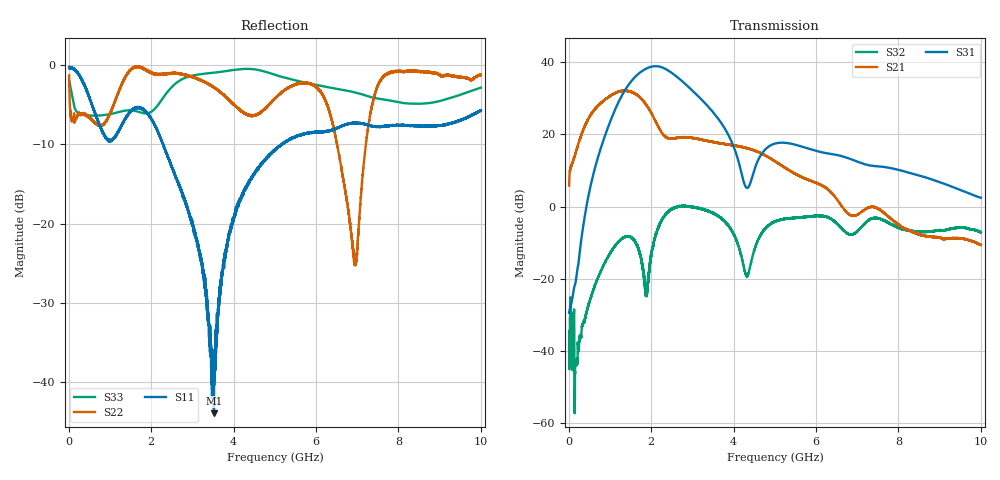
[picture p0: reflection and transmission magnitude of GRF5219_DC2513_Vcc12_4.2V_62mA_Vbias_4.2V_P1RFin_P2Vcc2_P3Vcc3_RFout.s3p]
!Keysight Technologies,N5245B,MY56052315,A.20.20.05
!Date: Friday, August 21, 2026 15:38:49
!Correction: S11(C  3-Port  )
!S12(C  3-Port  )
!S13(C  3-Port  )
!S21(C  3-Port  )
!S22(C  3-Port  )
!S23(C  3-Port  )
!S31(C  3-Port  )
!S32(C  3-Port  )
!S33(C  3-Port  )
!S3P File: Measurements: <S11,S12,S13>,
!<S21,S22,S23>,
!<S31,S32,S33>:
# Hz S  dB  R 50
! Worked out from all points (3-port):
!   9991 points, 10 MHz to 10 GHz, reference 50 ohm
!   strongest paths, dB at 10 MHz, 2.507 GHz, 5.005 GHz, 7.503 GHz, 10 GHz:
!     S31: -29.5, 37.0, 17.4, 11.1, 2.4
!     S21: 5.8, 18.8, 12.5, -0.6, -10.6
!     S32: -39.1, -0.7, -4.1, -3.2, -7.2
!   lowest |S11| = -43.9 dB at 3.524 GHz (marker M1), VSWR 1.01, Z = 49.9 - j0.623 ohm
!   |S11| at or under -10 dB: 2.290023 GHz to 2.292511 GHz (2.488 MHz wide, 0.109 % of centre); 2.293 GHz to 5.161 GHz (2.867 GHz wide, 76.9 % of centre); 5.161129 GHz to 5.16885 GHz (7.721 MHz wide, 0.149 % of centre)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
1e7  -0.37 -2.0  -54.46 -16.0  -63.07 72.6
     5.79 74.4  -1.31 -49.6  -58.02 113.3
     -29.47 -170.9  -39.08 7.9  -1.92 -57.0
6.06e8  -5.67 -92.1  -41.03 102.5  -66.14 110.3
        26.48 26.3  -7.09 169.1  -43.30 -64.5
        9.32 5.3  -22.71 2.6  -6.38 -168.3
1.133e9  -9.10 -105.4  -38.08 84.7  -59.09 69.9
         31.43 -34.8  -4.50 -162.3  -32.98 -137.8
         27.06 -60.8  -10.78 -64.6  -6.03 -169.4
1.51e9  -5.84 -137.3  -35.70 88.7  -57.39 82.5
        31.79 -89.0  -0.56 -175.9  -29.26 165.5
        34.60 -127.9  -8.55 -127.0  -5.69 -171.0
1.89e9  -6.04 170.0  -33.41 80.3  -56.34 59.4
        28.01 -142.4  -0.70 158.2  -31.11 118.8
        38.28 162.3  -23.57 -109.2  -6.09 -167.1
2.251e9  -9.56 122.3  -33.12 75.9  -56.85 58.9
         20.62 -160.6  -1.14 143.8  -32.06 113.9
         38.62 97.3  -4.00 -95.3  -4.42 -158.5
2.686e9  -15.17 77.8  -32.63 82.3  -59.73 65.3
         19.08 -149.0  -1.09 131.5  -29.60 90.3
         35.39 33.0  0.01 -158.2  -1.97 -167.8
3.524e9  -43.88 -102.5  -28.79 88.9  -56.91 72.9
         17.86 -179.5  -2.78 130.3  -30.35 36.9
         25.84 -53.5  -1.90 122.5  -0.96 169.6
5.005e9  -10.75 158.5  -27.03 66.4  -53.80 92.6
         12.55 109.1  -4.22 117.7  -38.76 57.2
         17.44 -34.2  -4.10 133.9  -1.22 147.5
1e10  -5.71 105.1  -25.57 35.8  -54.83 14.5
      -10.63 57.9  -1.24 86.4  -29.77 -20.6
      2.45 122.4  -7.22 -40.7  -2.84 77.4
